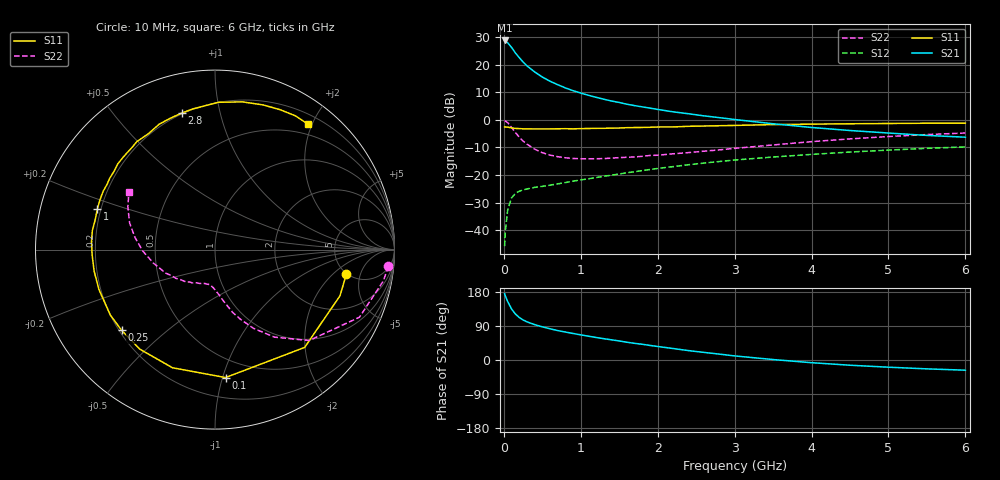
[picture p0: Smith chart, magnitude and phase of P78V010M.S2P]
! SIEMENS Small Signal Semiconductors
! BFP196
! Si NPN RF Bipolar Junction Transistor in SOT143
! VCE = 8 V  IC = 10 mA
! Common Emitter S-Parameters:  May  1996
# GHz  S  MA  R  50
!  f  S11  S21  S12  S22
! GHz  MAG  ANG  MAG  ANG  MAG  ANG  MAG  ANG
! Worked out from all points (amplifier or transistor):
!   36 points, 10 MHz to 6 GHz, reference 50 ohm
!   highest |S21| = 28.8 dB at 10 MHz (marker M1)
!   |S21| within 3 dB of that: start of sweep to 112.2 MHz
!   unconditionally stable (mu >= 1): 918.6 MHz to 3.334 GHz
!   at 250 MHz: K = 0.39, MSG = 23.2 dB, |S12| = -25.4 dB
!   at 1.4 GHz: K = 1.13, MAG = 11.2 dB, |S12| = -20.1 dB
!   at 6 GHz: K = 0.96, MSG = 1.8 dB, |S12| = -9.8 dB
!   S11 on the Smith chart (normalised r, x): 10 MHz: 4.97, -3.00; 100 MHz: 0.35, -1.02; 250 MHz: 0.21, -0.36; 1 GHz: 0.19, +0.16; 2.8 GHz: 0.20, +0.77; 6 GHz: 0.34, +1.94
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0.01  0.7446 -10.4  27.65 175.2  0.0051 89.6  0.9701 -5.5
0.02  0.7425 -20.3  26.84 168.8  0.0098 78.2  0.9544 -10.5
0.05  0.7392 -47.5  25.11 154.2  0.0231 67.9  0.8885 -25.1
0.1  0.7153 -85.3  20.7 134.8  0.0383 52.2  0.7292 -44.0
0.15  0.6996 -109.8  16.43 121.4  0.0463 42.9  0.5898 -55.8
0.2  0.6951 -127.1  13.52 112.3  0.0506 37.7  0.4878 -64.0
0.25  0.6877 -139.2  11.23 105.6  0.0536 34.9  0.4121 -70.0
0.3  0.6878 -148.0  9.591 100.8  0.0557 33.7  0.3634 -74.3
0.4  0.6839 -161.0  7.424 93.4  0.0595 32.7  0.2946 -80.2
0.5  0.684 -169.9  5.993 87.5  0.0621 33.7  0.2535 -84.8
0.6  0.6852 -177.5  5.037 82.4  0.0653 34.8  0.2297 -88.8
0.7  0.6897 176.2  4.35 77.6  0.0689 36.1  0.2147 -92.0
0.8  0.6915 171.2  3.806 73.8  0.0728 37.1  0.2052 -95.1
1  0.6933 161.0  3.067 66.3  0.0813 39.6  0.1971 -100.5
1.1  0.698 156.9  2.794 62.8  0.0852 40.7  0.1968 -103.4
1.6  0.7221 138.7  1.925 46.9  0.1095 43.0  0.2096 -116.9
2.2  0.7443 120.0  1.4 30.3  0.1418 41.6  0.2424 -132.2
2.8  0.7832 103.6  1.099 15.6  0.1754 37.4  0.2853 -149.9
3.5  0.821 88.6  0.85 1.2  0.2118 30.5  0.3508 -167.5
4.5  0.8496 71.5  0.641 -13.8  0.2607 20.0  0.4517 171.2
5.5  0.8698 58.9  0.522 -23.4  0.3042 8.9  0.5408 153.9
6  0.8697 53.4  0.485 -26.9  0.3237 2.7  0.5782 146.0
